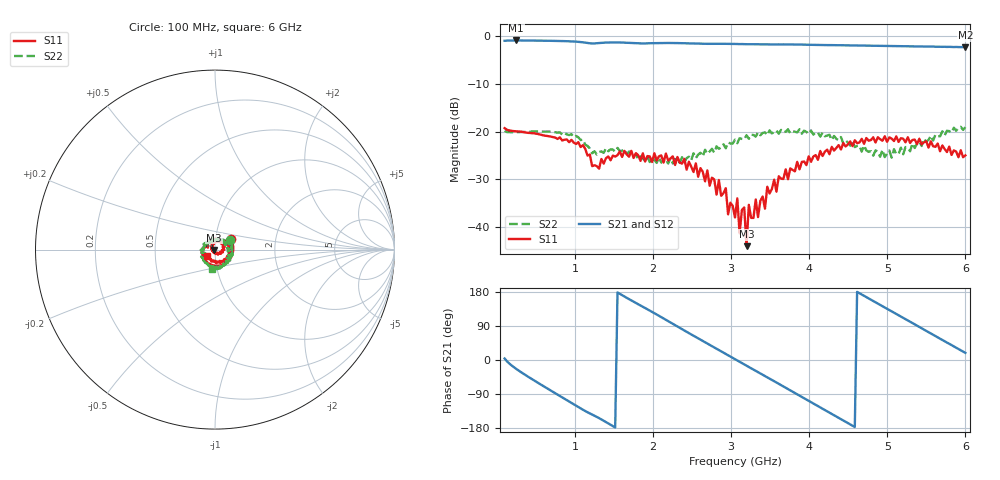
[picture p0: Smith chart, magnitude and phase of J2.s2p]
!Agilent Technologies,E8364B,MY43040379,A.07.50.67
!Agilent E8364B: A.07.50.67
!Date: Tuesday, March 24, 2026 11:35:57
!Correction: S11(Full 2 Port(1,2))
!S21(Full 2 Port(1,2))
!S12(Full 2 Port(1,2))
!S22(Full 2 Port(1,2))
!S2P File: Measurements: S11, S21, S12, S22:
# Hz S  dB  R 50
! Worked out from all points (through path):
!   201 points, 100 MHz to 6 GHz, reference 50 ohm
!   highest |S21| = -0.98 dB at 247.5 MHz (marker M1); lowest = -2.4 dB at 6 GHz (marker M2)
!   group delay of S21, straight-line fit = 326 ps
!   lowest |S11| = -43.9 dB at 3.197 GHz (marker M3), VSWR 1.01, Z = 49.4 - j0.263 ohm
!   |S11| at or under -10 dB: start of sweep to end of sweep
!   |S22| runs from -26.7 to -19.0 dB; largest |S21 - S12| = 0.0027
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1e8  -19.29 34.2  -1.05 4.0  -1.05 3.9  -19.88 33.5
2.475e8  -19.95 -15.3  -0.98 -23.3  -0.99 -23.4  -20.11 -10.7
6.9e8  -21.05 -95.3  -1.06 -80.5  -1.06 -80.6  -20.01 -79.0
1.103e9  -22.85 179.9  -1.37 -131.2  -1.37 -131.4  -21.68 -145.2
1.3095e9  -27.76 164.9  -1.53 -153.3  -1.52 -153.4  -24.28 -152.8
1.5455e9  -24.93 126.3  -1.39 178.3  -1.39 178.2  -23.43 176.0
2.0765e9  -25.17 48.5  -1.52 116.6  -1.52 116.5  -25.43 115.1
2.519e9  -28.46 -7.3  -1.64 64.1  -1.64 63.9  -24.55 84.8
2.8435e9  -30.13 -58.1  -1.68 26.5  -1.68 26.4  -23.61 50.4
3.05e9  -37.96 -85.6  -1.71 2.3  -1.71 2.2  -21.70 33.6
3.0795e9  -33.97 -110.9  -1.72 -1.2  -1.72 -1.3  -22.45 30.0
3.109e9  -41.26 -140.7  -1.75 -4.7  -1.74 -4.8  -21.40 31.5
3.168e9  -35.87 -153.1  -1.76 -11.6  -1.76 -11.6  -21.65 23.6
3.1975e9  -43.95 -155.2  -1.77 -15.0  -1.77 -15.1  -20.77 18.1
3.227e9  -35.30 -146.6  -1.77 -18.4  -1.78 -18.5  -21.52 12.6
3.345e9  -37.87 145.0  -1.81 -32.0  -1.81 -32.0  -20.15 1.1
3.6695e9  -29.92 119.6  -1.80 -69.9  -1.80 -69.9  -20.14 -44.5
4.053e9  -25.22 78.1  -1.90 -114.9  -1.90 -114.9  -20.65 -97.2
4.5545e9  -23.04 30.5  -2.01 -173.4  -2.02 -173.4  -21.96 -178.1
5.0265e9  -21.22 -8.8  -2.17 131.8  -2.16 131.8  -23.97 74.6
5.4985e9  -22.03 -66.1  -2.24 76.9  -2.24 76.8  -22.12 -23.1
6e9  -24.98 -143.3  -2.38 18.8  -2.38 18.8  -19.08 -97.7
